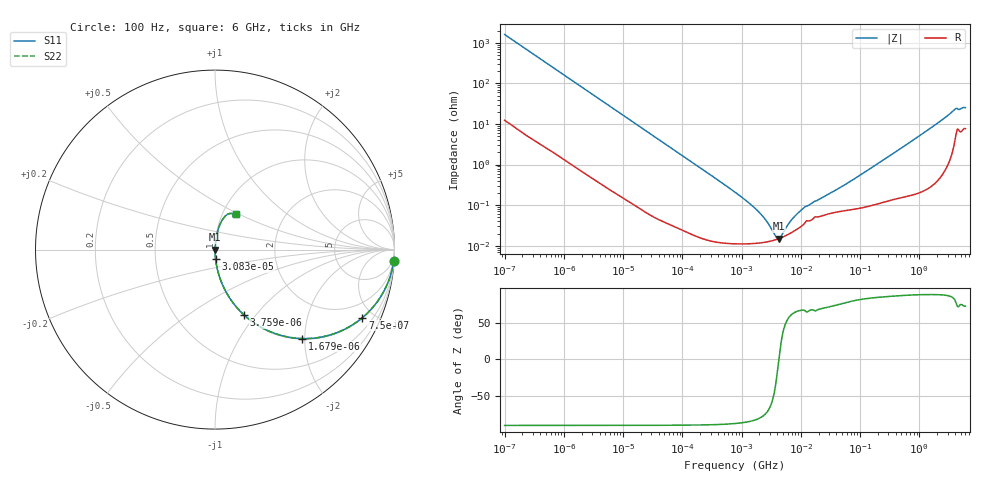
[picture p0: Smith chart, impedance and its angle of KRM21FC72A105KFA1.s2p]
!Murata Part Number: KRM21FC72A105KFA1
!These Parameters are Measured in Series Mode Connection
!Data Generated on Jan 08, 2026
!  o--ll--o
!Port1  Port2
!  o------o
!Operation Temp=25[degC], DC Bias Voltage=0[V]
!Freq. Start=100[Hz] Stop=6[GHz] 401[Steps]
# Hz S RI R 50
!Freq.(Hz) S11(Real) S11(Imag) S21(Real) S21(Imag) S12(Real) S12(Imag) S22(Real) S22(Imag)
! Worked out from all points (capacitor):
!   401 points, 100 Hz to 6 GHz, reference 50 ohm
!   read as one part in series: C = 990 nF near 109 Hz
!   lowest |Z| = 15 mohm at 4.246 MHz (marker M1)
!   series resonance near 4.256 MHz, so ESL is about 1.4 nH
!   S11 on the Smith chart (normalised r, x): 100 Hz: 1, -32; 750 Hz: 1.04, -4.32; 1.679 kHz: 1.02, -1.94; 3.759 kHz: 1.01, -0.87; 30.83 kHz: 1.00, -0.11; 6 GHz: 1.15, +0.48
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100  0.9957 -0.062  0.00434 0.062  0.00434 0.062  0.9957 -0.062
350  0.9535 -0.2066  0.0465 0.2066  0.0465 0.2066  0.9535 -0.2066
750  0.8216 -0.3788  0.1784 0.3788  0.1784 0.3788  0.8216 -0.3788
1679  0.4845 -0.4956  0.5155 0.4956  0.5155 0.4956  0.4845 -0.4956
2008  0.3976 -0.4852  0.6024 0.4852  0.6024 0.4852  0.3976 -0.4852
3759  0.1611 -0.3634  0.8389 0.3634  0.8389 0.3634  0.1611 -0.3634
8047  0.0415 -0.1951  0.9585 0.1951  0.9585 0.1951  0.0415 -0.1951
30832  0.0034 -0.0534  0.9966 0.0534  0.9966 0.0534  0.0034 -0.0534
40335  0.00212 -0.0409  0.9979 0.0409  0.9979 0.0409  0.00212 -0.0409
774597  0.000116 -0.00209  0.9999 0.00209  0.9999 0.00209  0.000116 -0.00209
1983483  0.000117 -0.000657  0.9999 0.000657  0.9999 0.000657  0.000117 -0.000657
2713602  0.000125 -0.000362  0.9999 0.000362  0.9999 0.000362  0.000125 -0.000362
3712478  0.00014 -0.000106  0.9999 0.000106  0.9999 0.000106  0.00014 -0.000106
4246196  0.00015 -1.7e-06  0.9999 1.7e-06  0.9999 1.7e-06  0.00015 -1.7e-06
7947587  0.000237 0.000485  0.9998 -0.000485  0.9998 -0.000485  0.000237 0.000485
1.137099e7  0.000348 0.000802  0.9997 -0.000802  0.9997 -0.000802  0.000348 0.000802
1.555665e7  0.000444 0.00105  0.9996 -0.00105  0.9996 -0.00105  0.000444 0.00105
5.699437e7  0.000746 0.00318  0.9993 -0.00318  0.9993 -0.00318  0.000746 0.00318
3.124326e8  0.00156 0.0162  0.9984 -0.0162  0.9984 -0.0162  0.00156 0.0162
1.369159e9  0.00732 0.0692  0.9927 -0.0692  0.9927 -0.0692  0.00732 0.0692
3.8344e9  0.0691 0.1959  0.9309 -0.1959  0.9309 -0.1959  0.0691 0.1959
6e9  0.1154 0.1974  0.8846 -0.1974  0.8846 -0.1974  0.1154 0.1974
